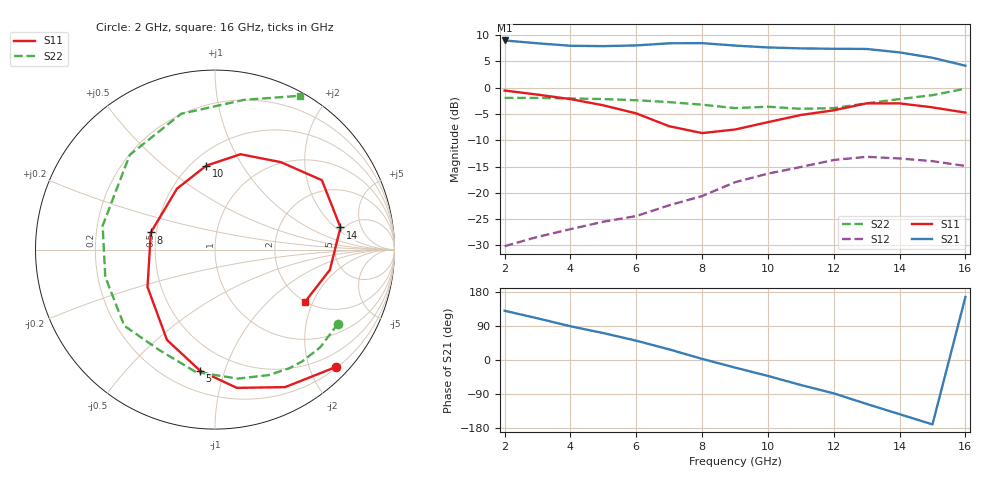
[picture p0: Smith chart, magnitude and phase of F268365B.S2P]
!ATF-26836
!S-PARAMETERS at Vds=5V  Id=30mA.  LAST UPDATED 07-22-92
# ghz s ma r 50
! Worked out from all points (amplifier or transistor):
!   15 points, 2 GHz to 16 GHz, reference 50 ohm
!   highest |S21| = 9.0 dB at 2 GHz (marker M1)
!   |S21| within 3 dB of that: start of sweep to 14.71 GHz
!   unconditionally stable (mu >= 1): nowhere
!   at 4 GHz: K = 0.72, MSG = 17.5 dB, |S12| = -26.9 dB
!   at 9 GHz: K = 0.69, MSG = 13.0 dB, |S12| = -18.0 dB
!   at 16 GHz: K = -0.23, MSG = 9.5 dB, |S12| = -14.9 dB
!   S11 on the Smith chart (normalised r, x): 2 GHz: 0.22, -2.46; 5 GHz: 0.33, -0.83; 8 GHz: 0.47, +0.10; 10 GHz: 0.59, +0.71; 14 GHz: 4.69, +2.33; 16 GHz: 2.00, -1.75
2  0.94 -44.0  2.82 130.0  0.031 65.0  0.8 -31.0
3  0.86 -63.0  2.65 110.0  0.038 56.0  0.8 -43.0
4  0.78 -81.0  2.51 89.0  0.045 47.0  0.79 -52.0
5  0.68 -97.0  2.49 71.0  0.053 41.0  0.78 -58.0
6  0.57 -118.0  2.53 51.0  0.06 39.0  0.76 -67.0
7  0.43 -151.0  2.65 28.0  0.076 38.0  0.73 -80.0
8  0.37 165.0  2.66 3.0  0.093 30.0  0.69 -99.0
9  0.4 122.0  2.52 -20.0  0.126 15.0  0.64 -119.0
10  0.47 96.0  2.42 -42.0  0.152 3.0  0.66 -140.0
11  0.55 75.0  2.37 -66.0  0.176 -4.0  0.63 -166.0
12  0.61 53.0  2.35 -88.0  0.205 -19.0  0.64 168.0
13  0.71 33.0  2.34 -116.0  0.22 -39.0  0.71 132.0
14  0.71 10.0  2.17 -143.0  0.212 -56.0  0.78 104.0
15  0.65 -10.0  1.93 -170.0  0.2 -72.0  0.85 79.0
16  0.58 -30.0  1.62 166.0  0.18 -93.0  0.98 61.0
